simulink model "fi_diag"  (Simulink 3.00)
settings: Solver=ode45  SolverMode=SingleTasking  StartTime=0.0  StopTime=10  MaxStep=st_size  RelTol=1e-5  AbsTol=1e-6
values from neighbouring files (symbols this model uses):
  d_through_p = get(MAIN_MENU(19),'Value')    [cback.m]    (also in imcmenu.m = 0)
  Disturb = Setpoint    [mimo_MSF1DF_sim.m]    (also in mimo_MSF2DF_sim.m)
  Satlb = temp1    [cback.m]    (also in imcmenu.m = str2num(satlbs))
  Satub = temp1    [cback.m]    (also in imcmenu.m = str2num(satubs))
  Setpoint = zeros(1,n)    [mimo_MSF1DF_sim.m]    (also in mimo_MSF2DF_sim.m)
undefined symbols (not defined in the file or in its folder): denPd, denPs, KI, numPd, numPs, Pre_fil_den, Pre_fil_num
libraries: MIMO_lib x1

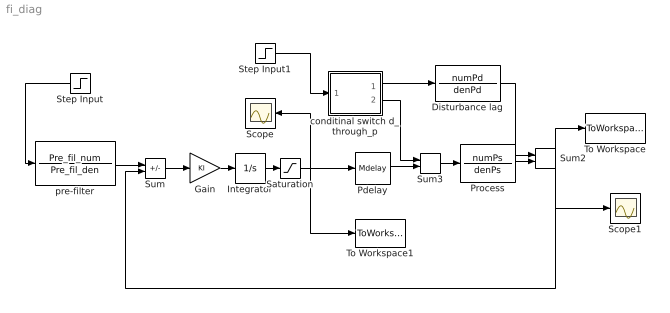
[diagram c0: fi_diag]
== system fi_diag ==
  Disturbance lag : TransferFcn  Numerator=numPd  Denominator=denPd
  Gain : Gain  Gain=KI  SaturateOnIntegerOverflow=on
  Integrator : Integrator  ExternalReset=none  InitialConditionSource=internal  InitialCondition=0  LimitOutput=off  UpperSaturationLimit=inf  LowerSaturationLimit=-inf  ShowSaturationPort=off  ShowStatePort=off  AbsoluteTolerance=auto
  Pdelay : MIMO_lib/Mdelay  Mdelay=Pdelay
  Process : TransferFcn  Numerator=numPs  Denominator=denPs
  Saturation : Saturate  UpperLimit=Satub  LowerLimit=Satlb
  Scope : Scope
  Scope1 : Scope
  Step Input : Step  Orientation=left  Time=0  Before=0  After=Setpoint  SampleTime=0
  Step Input1 : Step  Time=0  Before=0  After=Disturb  SampleTime=0
  Sum : Sum  Inputs=+-  SaturateOnIntegerOverflow=on
  Sum2 : Sum  Inputs=++  SaturateOnIntegerOverflow=on
  Sum3 : Sum  Inputs=++  SaturateOnIntegerOverflow=on
  To Workspace : ToWorkspace  VariableName=simout  SampleTime=-1  SaveFormat=Matrix
  To Workspace1 : ToWorkspace  VariableName=effort  SampleTime=-1  SaveFormat=Matrix
  conditinal switch d_through_p : Subsystem  Description=pass input signal through out1 if condition is true.
  pre-filter : TransferFcn  Numerator=Pre_fil_num  Denominator=Pre_fil_den
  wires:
  Step Input/1 -> pre-filter/1
  pre-filter/1 -> Sum/1
  Integrator/1 -> Saturation/1
  Gain/1 -> Integrator/1
  Sum/1 -> Gain/1
  conditinal switch d_through_p/1(Out2) -> Disturbance lag/1
  Disturbance lag/1 -> Sum2/1
  Pdelay/1 -> Sum3/2
  conditinal switch d_through_p/2(Out1) -> Sum3/1
  Sum3/1 -> Process/1
  Process/1 -> Sum2/2
  Step Input1/1 -> conditinal switch d_through_p/1(In)
  Saturation/1 -> Pdelay/1, Scope/1, To Workspace1/1
  Sum2/1 -> Sum/2, To Workspace/1, Scope1/1

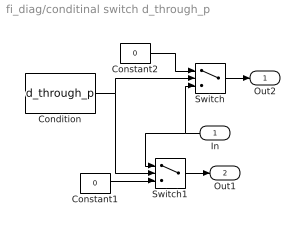
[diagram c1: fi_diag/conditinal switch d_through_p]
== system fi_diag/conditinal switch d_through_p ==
  In : Inport  Orientation=left  Port=1  PortWidth=-1  SampleTime=-1  DataType=auto
  Condition : Constant  Value=d_through_p
  Constant1 : Constant  Value=0
  Constant2 : Constant  Value=0
  Switch : Switch  Threshold=1
  Switch1 : Switch  Threshold=1
  Out2 : Outport  Port=1  InitialOutput=0
  Out1 : Outport  Port=2  InitialOutput=0
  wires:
  In/1 -> Switch/3, Switch1/1
  Condition/1 -> Switch1/2, Switch/2
  Constant1/1 -> Switch1/3
  Constant2/1 -> Switch/1
  Switch/1 -> Out2/1
  Switch1/1 -> Out1/1
